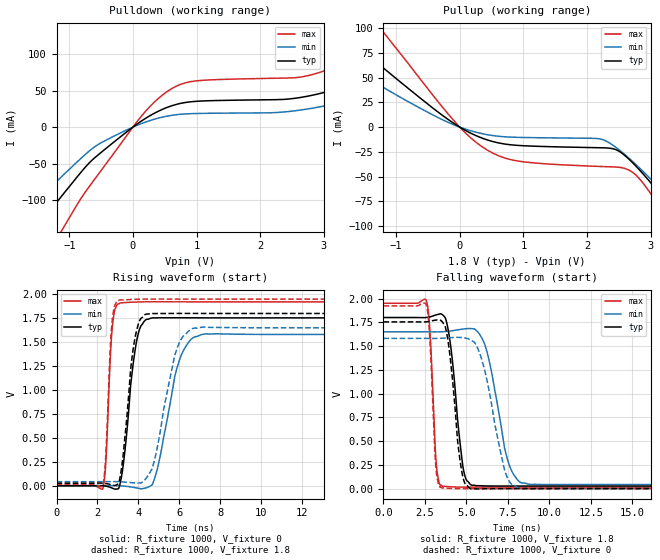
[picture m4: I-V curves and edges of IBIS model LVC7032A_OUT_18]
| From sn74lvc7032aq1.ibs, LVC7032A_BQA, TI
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[Model]   LVC7032A_OUT_18
Model_type  Output
Vref =   0
Rref =   1000
Cref =   30p
Vmeas =   0.9
| variable   typ   min   max
C_comp   6.70pF   4.39pF   9.98pF
| C_pullup   5.88pF   4.39pF   6.79pF
| C_pulldown   7.51pF   4.67pF   9.98pF
[Temperature Range]   40   100   -40
| Ambient temperature   25   85   -40
[Voltage range]   1.8   1.65   1.95
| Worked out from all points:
|   slope of the pulldown table from 0 to 0.27 V, typ, clamps not added: 17.1 ohm
|   slope of the pullup table from 0 to 0.27 V, typ, clamps not added: 29.9 ohm
|   rising waveform, R_fixture 1000, V_fixture 0: 20-80 % time 497ps typ, 864ps min, 238ps max; typ from 0 V to 1.75 V
|   falling waveform, R_fixture 1000, V_fixture 1.8: 20-80 % time 592ps typ, 995ps min, 295ps max; typ from 1.8 V to 0.027 V
|   rising waveform, R_fixture 1000, V_fixture 1.8: 20-80 % time 474ps typ, 856ps min, 233ps max; typ from 0.027 V to 1.8 V
|   falling waveform, R_fixture 1000, V_fixture 0: 20-80 % time 569ps typ, 1.07ns min, 293ps max; typ from 1.75 V to 0 V
[Pulldown]
| LVC7032A_OUT_18
|   Voltage   I(typ)   I(min)   I(max)
-5.5V     -559.1mA   -452.2mA   -710.9mA
-2.18V    -208.5mA   -158.8mA   -285.4mA
-1.865V   -175.2mA   -131.6mA   -244.5mA
-1.48V    -133.9mA   -98.56mA   -193.1mA
-1.07V    -89.31mA   -63.76mA   -134.9mA
70mV      4.491mA    2.617mA    8.125mA
615mV     29.45mA    16.27mA    53.12mA
2.815V    43.69mA    25.92mA    72.1mA
4.325V    93.52mA    64.21mA    142.7mA
5.155V    134.5mA    96.03mA    199.6mA
6.155V    191.3mA    141.3mA    276.1mA
11V       510.2mA    405.2mA    689.3mA
[Pullup]
| LVC7032A_OUT_18
|   Voltage   I(typ)   I(min)   I(max)
-5.5V     324.9mA    249.5mA    454.8mA
-2.68V    143.9mA    103mA      216.3mA
-2.015V   104.9mA    73.15mA    161.8mA
-1.32V    66.21mA    44.72mA    105.6mA
360mV     -11.3mA    -6.711mA   -20.18mA
985mV     -18.72mA   -10.42mA   -34.9mA
2.465V    -23.02mA   -20.97mA   -40.36mA
2.785V    -40.46mA   -38.76mA   -49.43mA
3.365V    -85.63mA   -77.45mA   -103.2mA
3.56V     -102.6mA   -91.66mA   -124.4mA
3.775V    -122mA     -107.8mA   -148.7mA
11V       -874.4mA   -739.7mA   -1.068A
[Ramp]
| LVC7032A_OUT_18
| variable   typ   min   max
dV/dt_r   1.07/5.23E-10   0.97/9.95E-10   1.17/2.59E-10
dV/dt_f   1.09/6.29E-10   0.98/1.11E-09   1.19/3.14E-10
R_load = 1000
[Rising Waveform]
| LVC7032A_OUT_18
R_fixture =   1000
C_fixture =   0
L_fixture =   0
V_fixture =   0
V_fixture_min = 0
V_fixture_max = 0
|   Time   V(typ)   V(min)   V(max)
0s        194.2pV    4.892nV    16.26pV
2.265ns   -225.2uV   331.2uV    -33.36mV
2.415ns   -4.693mV   537.6uV    261.5mV
2.725ns   -24.78mV   768uV      1.651V
3.11ns    21.97mV    -805.1uV   1.909V
3.87ns    1.454V     -21.08mV   1.92V
4.405ns   1.739V     -20.56mV   1.922V
5.97ns    1.755V     1.286V     1.922V
6.765ns   1.755V     1.556V     1.922V
24.99ns   1.754V     1.581V     1.922V
[Falling Waveform]
| LVC7032A_OUT_18
R_fixture =   1000
C_fixture =   0
L_fixture =   0
V_fixture =   1.8
V_fixture_min = 1.65
V_fixture_max = 1.95
|   Time   V(typ)   V(min)   V(max)
0s        1.8V       1.65V      1.95V
2.605ns   1.801V     1.65V      1.968V
3.19ns    1.828V     1.649V     259mV
3.565ns   1.829V     1.651V     24.15mV
4.045ns   1.514V     1.658V     19.5mV
4.79ns    234.7mV    1.678V     15.85mV
5.295ns   37.31mV    1.684V     15.78mV
6.12ns    28.65mV    1.514V     16.11mV
8.28ns    27.01mV    63.57mV    16.27mV
24.99ns   27.13mV    42.42mV    16.27mV
[Rising Waveform]
| LVC7032A_OUT_18
R_fixture =   1000
C_fixture =   0
L_fixture =   0
V_fixture =   1.8
V_fixture_min = 1.65
V_fixture_max = 1.95
|   Time   V(typ)   V(min)   V(max)
0s        27.13mV    42.42mV    16.27mV
2.26ns    26.9mV     42.69mV    -7.067mV
2.41ns    23.12mV    42.83mV    321.1mV
2.695ns   8.939mV    42.87mV    1.659V
2.995ns   17.28mV    42.07mV    1.936V
3.795ns   1.491V     30.45mV    1.948V
4.37ns    1.793V     73.48mV    1.95V
5.82ns    1.801V     1.388V     1.95V
6.665ns   1.8V       1.643V     1.95V
24.99ns   1.8V       1.65V      1.95V
[Falling Waveform]
| LVC7032A_OUT_18
R_fixture =   1000
C_fixture =   0
L_fixture =   0
V_fixture =   0
V_fixture_min = 0
V_fixture_max = 0
|   Time   V(typ)   V(min)   V(max)
0s        1.754V     1.581V     1.922V
2.59ns    1.755V     1.581V     1.927V
2.805ns   1.76V      1.58V      1.557V
3.145ns   1.773V     1.58V      269mV
3.4ns     1.773V     1.581V     16.24mV
3.915ns   1.532V     1.586V     3.96mV
4.735ns   170.4mV    1.589V     -389.3uV
5.255ns   -2.051mV   1.565V     -466.1uV
8.13ns    -93.44uV   5.975mV    1.077uV
24.99ns   9.595nV    25.78nV    8.987nV
